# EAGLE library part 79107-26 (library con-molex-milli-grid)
RECEPTACAL
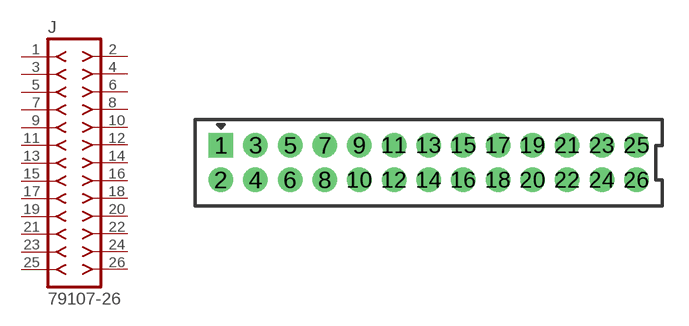
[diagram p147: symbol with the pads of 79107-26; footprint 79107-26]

Designator prefix J

## 79107-26  [79107-26]
1  1  pas
2  2  pas
3  3  pas
4  4  pas
5  5  pas
6  6  pas
7  7  pas
8  8  pas
9  9  pas
10  10  pas
11  11  pas
12  12  pas
13  13  pas
14  14  pas
15  15  pas
16  16  pas
17  17  pas
18  18  pas
19  19  pas
20  20  pas
21  21  pas
22  22  pas
23  23  pas
24  24  pas
25  25  pas
26  26  pas

## Footprint 79107-26 (pad centres in mm)
RECEPTACAL Dual Row, Vertical, Through-Hole
drill 0.914 square: 1 -12,1
drill 0.914: 2 -12,-1; 3 -10,1; 4 -10,-1; 5 -8,1; 6 -8,-1; 7 -6,1; 8 -6,-1; 9 -4,1; 10 -4,-1; 11 -2,1; 12 -2,-1; 13 0,1; 14 0,-1; 15 2,1; 16 2,-1; 17 4,1; 18 4,-1; 19 6,1; 20 6,-1; 21 8,1; 22 8,-1; 23 10,1; 24 10,-1; 25 12,1; 26 12,-1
